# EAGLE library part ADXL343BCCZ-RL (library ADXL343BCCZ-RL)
Accelerometer X, Y, Z Axis +/-2g, 4g, 8g, 16g 0.05Hz ~ 1.6kHz 14-LGA (3x5) Source: Datasheet
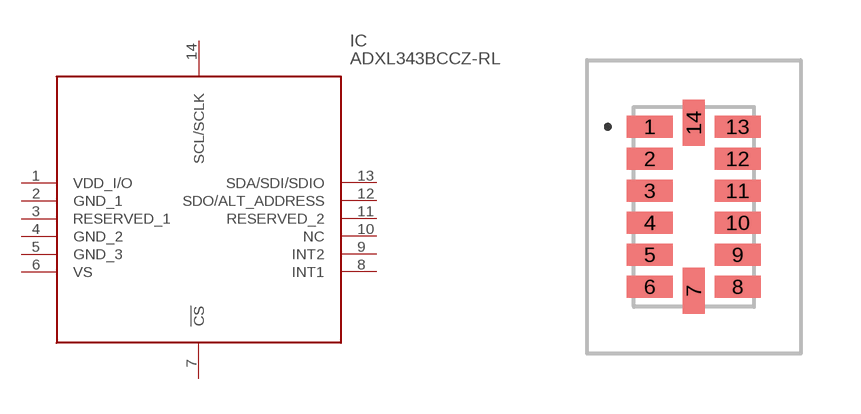
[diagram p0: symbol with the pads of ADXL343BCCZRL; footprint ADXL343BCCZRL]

Designator prefix IC

## ADXL343BCCZ-RL (Arrow_Part_Number: ADXL343BCCZ-RL; Arrow_Price-Stock: https://www.arrow.com/en/products/adxl343bccz-rl/analog-devices?region=nac; Description: Accelerometer X, Y, Z Axis +/-2g, 4g, 8g, 16g 0.05Hz ~ 1.6kHz 14-LGA (3x5); Height: 1mm; Manufacturer_Name: Analog Devices; Manufacturer_Part_Number: ADXL343BCCZ-RL; Mouser_Part_Number: 584-ADXL343BCCZ-R; Mouser_Price-Stock: https://www.mouser.co.uk/ProductDetail/Analog-Devices/ADXL343BCCZ-RL?qs=WIvQP4zGaniHpowyrbt1Aw%3D%3D)  [ADXL343BCCZRL]
1  VDD_I/O
2  GND_1
3  RESERVED_1
4  GND_2
5  GND_3
6  VS
7  !CS
8  INT1
9  INT2
10  NC  nc
11  RESERVED_2
12  SDO/ALT_ADDRESS
13  SDA/SDI/SDIO
14  SCL/SCLK

## Footprint ADXL343BCCZRL (pad centres in mm)
14-Terminal Land Grid Array [LGA] (CC-14-1)
smd 1.145 x 0.55: 1 -1.098,2; 2 -1.098,1.2; 3 -1.098,0.4; 4 -1.098,-0.4; 5 -1.098,-1.2; 6 -1.098,-2; 8 1.098,-2; 9 1.098,-1.2; 10 1.098,-0.4; 11 1.098,0.4; 12 1.098,1.2; 13 1.098,2
smd 0.55 x 1.145: 7 0,-2.098; 14 0,2.098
